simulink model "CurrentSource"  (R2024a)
settings: Solver=VariableStepAuto  StartTime=0.0  StopTime=1e-5  RelTol=1e-3  AbsTol=1e-3
libraries: fl_lib x10, nesl_utility x3, ee_lib x2

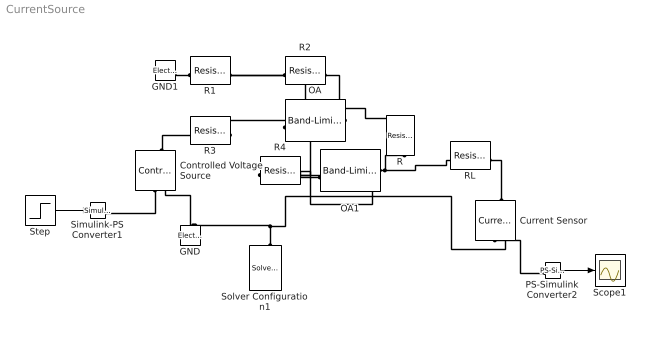
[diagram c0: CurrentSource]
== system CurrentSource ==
  Controlled Voltage Source : fl_lib/Electrical/Electrical Sources/Controlled Voltage Source
  Current Sensor : fl_lib/Electrical/Electrical Sensors/Current Sensor
  GND : fl_lib/Electrical/Electrical Elements/Electrical Reference
  GND1 : fl_lib/Electrical/Electrical Elements/Electrical Reference
  OA : ee_lib/Integrated Circuits/Band-Limited Op-Amp  A=1e6  Rin=1e6 Ohm  Rout=0 Ohm  Vmin=-15 V  Vmax=15 V  Vdotmax=1e7 V/s  f=5 Hz  V0=0 V
  OA1 : ee_lib/Integrated Circuits/Band-Limited Op-Amp  A=1e6  Rin=1e6 Ohm  Rout=0 Ohm  Vmin=-15 V  Vmax=15 V  Vdotmax=1e7 V/s  f=5 Hz  V0=0 V
  PS-Simulink Converter2 : nesl_utility/PS-Simulink Converter  PhysicalDomain=network_engine_domain  SubClassName=ps_output  LeftPortType=input  RightPortType=output  PseudoPeriodic=off  Frequencies=[]  VectorFormat=1-D array  Unit=inherit  AffineConversion=off
  R : fl_lib/Electrical/Electrical Elements/Resistor  R=2.5 kOhm  i_specify=off  i_priority=None  i=0 A  i_nominal_specify=off  i_nominal_value=1  i_nominal_unit=A  v_specify=off  v_priority=None  v=0 V  v_nominal_specify=off  v_nominal_value=1  v_nominal_unit=V
  R{1..4} (4 alike) : fl_lib/Electrical/Electrical Elements/Resistor  R=25 kOhm  i_specify=off  i_priority=None  i=0 A  i_nominal_specify=off  i_nominal_value=1  i_nominal_unit=A  v_specify=off  v_priority=None  v=0 V  v_nominal_specify=off  v_nominal_value=1  v_nominal_unit=V
  RL : fl_lib/Electrical/Electrical Elements/Resistor  R=100 Ohm  i_specify=off  i_priority=None  i=0 A  i_nominal_specify=off  i_nominal_value=1  i_nominal_unit=A  v_specify=off  v_priority=None  v=0 V  v_nominal_specify=off  v_nominal_value=1  v_nominal_unit=V
  Scope1 : Scope
  Simulink-PS Converter1 : nesl_utility/Simulink-PS Converter  PhysicalDomain=network_engine_domain  SubClassName=ps_input  LeftPortType=input  RightPortType=output  PseudoPeriodic=off  Frequencies=[]  NoiseDistribution=none  NoiseParameters=[]  Unit=1  AffineConversion=off  FilteringAndDerivatives=provide  SimscapeFilterOrder=1  InputFilterTimeConstant=0.001  UdotUserProvided=0
  Solver Configuration1 : nesl_utility/Solver Configuration  PhysicalDomain=network_engine_domain  SubClassName=solver  LeftPortType=input  RightPortType=generic  Tones=[]  Harmonics=[]  SimulateNoise=off  Profile=off  UseLocalSampling=off  EnableSwitchedLinearOptims=on  FrequencyDomain=off  UseCCode=off  RelTol=0.001  AbsTol=1e-06  MinStep=1e-09  ToWorkspace=off  RevertToSquareIcSolve=off  NumHomotopyIterations=100  PhasorMode=off  PhasorModeNumHarmonics=1  ConsistencySolver=NEWTON_FTOL  IndexReductionMethod=DerivativeReplacement  DoDC=on  ResidualTolerance=1e-09  ConsistencyTolSource=GLOBAL  ConsistencyAbsTol=0.001  ConsistencyRelTol=0.001  ConsistencyTolFactor=0.001  UseLocalSolver=off  LocalSolverChoice=NE_BACKWARD_EULER_ADVANCER  ResolveIndetEquations=on  FunctionEvalNumThread=1  LocalSolverSampleTime=0.001  DoFixedCost=off  MaxNonlinIter=3  MaxModeIter=2  ComputeImpulses=off  ImpulseIterations=2  LinearAlgebra=Sparse  LinearAlgebraNumThread=0  EquationFormulation=NE_TIME_EF  DelaysMemoryBudget=1024  AutomaticFiltering=on  FilteringTimeConstant=0.001  PartitionStorageMethod=AS_NEEDED  PartitionMemoryBudget=1024  PartitionMethod=FAST  MultibodyUseLocalSolver=off  MultibodyLocalSolverChoice=ODE1  MultibodyLocalSolverSampleTime=0.001
  Step : Step  SampleTime=0
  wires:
  Step/1 -> Simulink-PS Converter1/1
  PS-Simulink Converter2/1 -> Scope1/1
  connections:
  Solver Configuration1/RConn1 -- Current Sensor/RConn2 -- GND/LConn1 -- Controlled Voltage Source/RConn2
  PS-Simulink Converter2/LConn1 -- Current Sensor/RConn1
  Controlled Voltage Source/RConn1 -- Simulink-PS Converter1/RConn1
  R2/LConn1 -- OA/RConn1 -- R/RConn1
  OA/LConn1 -- R4/RConn1 -- R3/LConn1
  R1/LConn1 -- OA/LConn2 -- R2/RConn1
  GND1/LConn1 -- R1/RConn1
  Controlled Voltage Source/LConn1 -- R3/RConn1
  OA1/RConn1 -- OA1/LConn2 -- R4/LConn1
  OA1/LConn1 -- RL/LConn1 -- R/LConn1
  Current Sensor/LConn1 -- RL/RConn1
